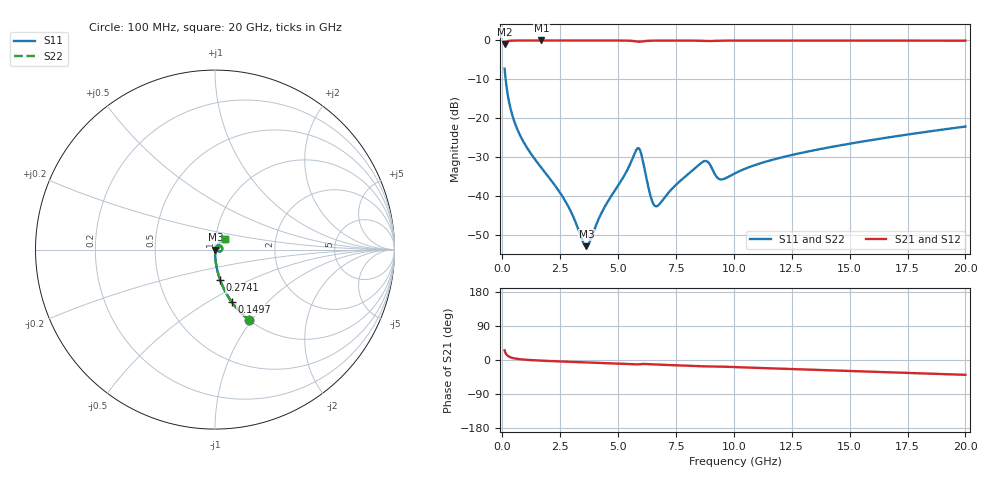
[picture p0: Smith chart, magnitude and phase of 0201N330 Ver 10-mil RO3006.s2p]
# GHz S MA R 50
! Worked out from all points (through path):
!   1601 points, 100 MHz to 20 GHz, reference 50 ohm
!   highest |S21| = -0.02 dB at 1.692 GHz (marker M1); lowest = -0.9 dB at 100 MHz (marker M2)
!   group delay of S21, straight-line fit = 5.8 ps
!   lowest |S11| = -53.0 dB at 3.632 GHz (marker M3), VSWR 1.00, Z = 50.2 - j0.0339 ohm
!   |S11| at or under -10 dB: 144.1 MHz to end of sweep
!   |S22| runs from -53.0 to -7.3 dB; largest |S21 - S12| = 0
!   S11 on the Smith chart (normalised r, x): 100 MHz: 1.00, -0.96; 149.8 MHz: 1.00, -0.64; 274.1 MHz: 1.00, -0.35; 20 GHz: 1.10, +0.13
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0.1  0.433 -64.4  0.9008 25.5  0.9008 25.5  0.433 -64.4
0.14975  0.3052 -72.4  0.9516 17.5  0.9516 17.5  0.3052 -72.4
0.274125  0.1719 -80.4  0.9844 9.4  0.9844 9.4  0.1719 -80.4
0.473125  0.09954 -84.7  0.9942 4.9  0.9942 4.9  0.09954 -84.7
0.74675  0.0618 -86.9  0.9971 2.2  0.9971 2.2  0.0618 -86.9
1.692  0.02282 -88.0  0.9982 -1.7  0.9982 -1.7  0.02282 -88.0
2.761625  0.00813 -81.1  0.998 -4.4  0.998 -4.4  0.00813 -81.1
3.420812  0.002839 -46.9  0.9978 -6.0  0.9978 -6.0  0.002839 -46.9
3.63225  0.002243 -8.7  0.9977 -6.4  0.9977 -6.4  0.002243 -8.7
4.366062  0.006689 57.9  0.9971 -8.1  0.9971 -8.1  0.006689 57.9
5.833687  0.04062 21.5  0.9656 -11.6  0.9656 -11.6  0.04062 21.5
6.007812  0.03385 -14.4  0.9661 -10.5  0.9661 -10.5  0.03385 -14.4
6.468  0.008589 -12.8  0.9912 -11.4  0.9912 -11.4  0.008589 -12.8
6.741625  0.007555 25.1  0.9938 -12.2  0.9938 -12.2  0.007555 25.1
7.487875  0.01372 56.2  0.9951 -14.0  0.9951 -14.0  0.01372 56.2
8.694313  0.02767 43.1  0.9856 -16.7  0.9856 -16.7  0.02767 43.1
8.90575  0.02672 29.1  0.981 -16.8  0.981 -16.8  0.02672 29.1
9.390812  0.01631 34.7  0.9896 -17.3  0.9896 -17.3  0.01631 34.7
10.05  0.01945 54.6  0.994 -18.8  0.994 -18.8  0.01945 54.6
13.37081  0.03801 57.7  0.9946 -25.6  0.9946 -25.6  0.03801 57.7
16.69162  0.05647 52.8  0.9932 -32.4  0.9932 -32.4  0.05647 52.8
20  0.07785 47.0  0.9912 -39.2  0.9912 -39.2  0.07785 47.0
